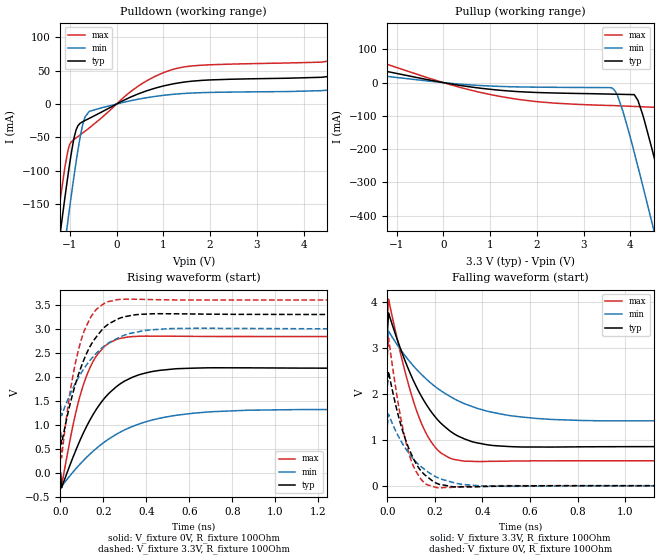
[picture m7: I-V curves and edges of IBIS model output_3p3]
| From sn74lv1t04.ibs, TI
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|   output_3p3 Model
[Model]   output_3p3
Model_type   Output
Polarity   Inverting
Vmeas = 1.65
Vref = 0
Cref = 30pF
Rref = 150
|   typ   min   max
|   (nom PVT)   (fast PVT)   (slow PVT)
C_comp   2.206e-12   2.118e-12   2.246e-12
| Where nom  PVT is Nominal Process, 3.3V, 40C
|   Fast PVT is Strong Process,  3.6V, -40C
|   Slow PVT is Weak Process,   3V, 140C
[Voltage Range]   3.3   3   3.6
|Junction Temperature
[Temperature Range]   40   140   -40
[Pullup Reference]   3.3   3   3.6
[Pulldown Reference]   0   0   0
[Power Clamp Reference]   3.3   3   3.6
[GND Clamp Reference]   0   0   0
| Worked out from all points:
|   slope of the pulldown table from 0 to 0.495 V, typ, clamps not added: 30.8 ohm
|   slope of the pullup table from 0 to 0.495 V, typ, clamps not added: 44 ohm
|   falling waveform, V_fixture 3.3V, R_fixture 100Ohm: 20-80 % time 161ps typ, 253ps min, 111ps max; typ from 3.3 V to 0.855 V
|   rising waveform, V_fixture 0V, R_fixture 100Ohm: 20-80 % time 179ps typ, 277ps min, 107ps max; typ from 0 V to 2.18 V
|   rising waveform, V_fixture 3.3V, R_fixture 100Ohm: 20-80 % time 123ps typ, 161ps min, 85.5ps max; typ from 0.855 V to 3.3 V
|   falling waveform, V_fixture 0V, R_fixture 100Ohm: 20-80 % time 90.4ps typ, 132ps min, 68.2ps max; typ from 2.18 V to 0 V
[Pulldown]
|   Voltage   I(typ)   I(min)   I(max)
-3.3V     -1.416A    -1.484A    -1.368A
-1.308V   -251.1mA   -322.1mA   -199.8mA
-1.19V    -186.2mA   -256.6mA   -136.5mA
-1.105V   -140.9mA   -210.2mA   -94.88mA
-1.036V   -105.4mA   -172.7mA   -68.28mA
-867.9mV  -39.39mA   -88.09mA   -50.95mA
-726mV    -26.58mA   -31.57mA   -43.59mA
-585mV    -21.58mA   -11.04mA   -35.97mA
458.4mV   15.09mA    7.21mA     26.68mA
1.194V    30.08mA    14.51mA    51.78mA
4.393V    40.23mA    20.15mA    62.96mA
6.6V      74.95mA    42.08mA    114.2mA
[Pullup]
|   Voltage   I(typ)   I(min)   I(max)
-3.3V     97.54mA    53.13mA    161.8mA
630.3mV   -13.91mA   -7.345mA   -24.17mA
3.58V     -34.56mA   -15.15mA   -68.93mA
3.726V    -35.01mA   -39.53mA   -69.57mA
4.083V    -36.21mA   -209.9mA   -71.7mA
4.264V    -96.36mA   -309.4mA   -72.77mA
4.478V    -208.3mA   -430.5mA   -74.05mA
4.591V    -271.1mA   -495.2mA   -94.92mA
4.839V    -412.1mA   -638.2mA   -221.5mA
5.103V    -564.8mA   -791.7mA   -371mA
5.646V    -882.6mA   -1.11A     -686.7mA
6.6V      -1.416A    -1.661A    -1.249A
[Ramp]
R_load = 100
|   typ   min   max
dV/dt_r   1.30763/1.78573e-10   0.786419/2.77202e-10   1.70433/1.06616e-10
dV/dt_f   1.46705/1.61002e-10   0.947458/2.52885e-10   1.83444/1.11129e-10
[Falling Waveform]
V_fixture = 3.3V
V_fixture_min = 3V
V_fixture_max = 3.6V
R_fixture = 100Ohm
|   Time   V(typ)   V(min)   V(max)
0s        3.3V       3V         3.6V
5ps       3.762V     3.366V     4.063V
90ps      2.522V     2.731V     2.185V
125ps     2.126V     2.522V     1.606V
160ps     1.801V     2.342V     1.172V
210ps     1.445V     2.124V     785.6mV
280ps     1.132V     1.896V     572.8mV
425ps     887.9mV    1.618V     530.7mV
690ps     841.8mV    1.443V     542.5mV
2.875ns   855mV      1.422V     542.5mV
[Rising Waveform]
V_fixture = 0V
V_fixture_min = 0V
V_fixture_max = 0V
R_fixture = 100Ohm
|   Time   V(typ)   V(min)   V(max)
0s        430.6pV    4.778nV    775.1pV
5ps       -309.6mV   -280.1mV   -270.8mV
50ps      231.2mV    -25.75mV   811.7mV
80ps      563.8mV    130.1mV    1.415V
135ps     1.083V     383.3mV    2.165V
200ps     1.53V      628.6mV    2.61V
280ps     1.861V     854.2mV    2.804V
465ps     2.138V     1.141V     2.849V
870ps     2.189V     1.306V     2.84V
3.01ns    2.179V     1.31V      2.841V
[Rising Waveform]
V_fixture = 3.3V
V_fixture_min = 3V
V_fixture_max = 3.6V
R_fixture = 100Ohm
|   Time   V(typ)   V(min)   V(max)
0s        854.9mV    1.421V     542.6mV
5ps       602.3mV    1.193V     317.3mV
50ps      1.527V     1.689V     1.819V
75ps      1.927V     1.913V     2.398V
100ps     2.252V     2.107V     2.818V
160ps     2.792V     2.458V     3.369V
220ps     3.089V     2.695V     3.563V
335ps     3.284V     2.916V     3.618V
510ps     3.314V     3.005V     3.603V
1.94ns    3.3V       2.999V     3.6V
[Falling Waveform]
V_fixture = 0V
V_fixture_min = 0V
V_fixture_max = 0V
R_fixture = 100Ohm
|   Time   V(typ)   V(min)   V(max)
0s        2.179V     1.311V     2.841V
5ps       2.488V     1.556V     3.221V
50ps      1.452V     1.042V     1.661V
75ps      1.024V     822.8mV    1.017V
95ps      759.3mV    675.2mV    632.1mV
135ps     366.6mV    445.6mV    191.9mV
170ps     189.6mV    303mV      15.8mV
265ps     -15.26mV   86.75mV    -37.34mV
405ps     -18.09mV   -6.878mV   -2.015mV
1.475ns   -36.83uV   620.4uV    -43.9uV
